(* Logix 5000 AddOnInstructionDefinition export; software revision 16.04 *)

TYPE AKD_Status :   // All connections to the drive ethernet module are established and data is successfully transferring.
STRUCT
   Profile_In_Progress : BOOL;   // Profile Move In Progress
   Block_In_Execution : BOOL;   // Block In Execution
   On_Target_Position : BOOL;   // On Target Position (1=Current Position Equals Last Target Position)
   General_Fault : BOOL;   // General Fault
   Current_Direction : BOOL;   // Current Motor Direction (0=Reverse, 1=Forward)
   Home_Level : BOOL;   // Level of Home Input
   Reg_Level : BOOL;   // Level of Registration Input
   Enable : BOOL;   // State of Enable Output
   Fault_Input_Fault : BOOL;   // Fault Input Active
   Fwd_Limit : BOOL;   // Forward Input Active
   Rev_Limit : BOOL;   // Reverse Input Active
   Positive_Limit : BOOL;   // Positive Software Limit Exceeded
   Negative_Limit : BOOL;   // Negative Software Limit Exceeded
   FE_Fault : BOOL;   // Following Error Fault
   Block_Fault : BOOL;   // Block Execution Fault
   Load_Complete : BOOL;   // Command Message Successfully Loaded
END_STRUCT
END_TYPE

TYPE AKD_Axis :   // Axis Data:
STRUCT
   Control : AKD_Control;   // Control bits to send to the drive
   Status : AKD_Status;   // Status bits received from the drive
   Input : AB:ETHERNET_MODULE_SINT_64Bytes:I:0;   // Data from the drive
   Output : AB:ETHERNET_MODULE_SINT_64Bytes:O:0;   // Data to the drive
   ResponseMsgType : SINT;   // Response type contained in latest IO response from drive. Used to check for errors
   CommandTimeout : INT;   // Time to allow for command response from drive. Dependent on scan rate and communicaiton rate
   PositionFeedback : DINT;   // Actual Position Value
   VelocityFeedback : DINT;   // Actual Velocity Value
END_STRUCT
END_TYPE

TYPE AKD_Control :   // Send Explicit Message
STRUCT
   Load_Data_Start_Profile : BOOL;   // Load Command Data / Start Profile Move
   Start_Block : BOOL;   // Execute Command block or block chain
   Incremental : BOOL;   // Incremental Position (0=Absolute, 1=Incremental)
   Direction : BOOL;   // Direction in Velocity Mode (0=Reverse, 1=Forward)
   Smooth_Stop : BOOL;   // Smooth / Controlled Stop w/ Deceleration
   Hard_Stop : BOOL;   // Hard / Immediate Stop
   Reg_Arm : BOOL;   // Arm the Registration Input
   Enable : BOOL;   // Enable Output
END_STRUCT
END_TYPE

ADD_ON_INSTRUCTION AKD_Disable   (* revision 2.1, ExecutePrescan, ExecuteEnableInFalse *)
// Disable Drive
// Revision note:
// Don't error if Command_Timeout preset is 0
VAR_OUTPUT
   DN : BOOL; {visible}   // Command Successful
   ER : BOOL; {visible}   // Error
END_VAR
VAR_IN_OUT
   Axis : AKD_Axis; {required}
END_VAR
VAR
   Command_Timeout : TIMER;   // Timeout Timer
END_VAR

ROUTINE EnableInFalse   (* ladder *)
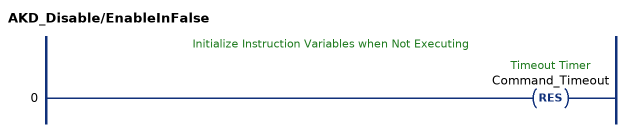
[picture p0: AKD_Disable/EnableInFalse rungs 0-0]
   // Initialize Instruction Variables when Not Executing
   0: RES(Command_Timeout);
END_ROUTINE

ROUTINE Logic   (* ladder *)
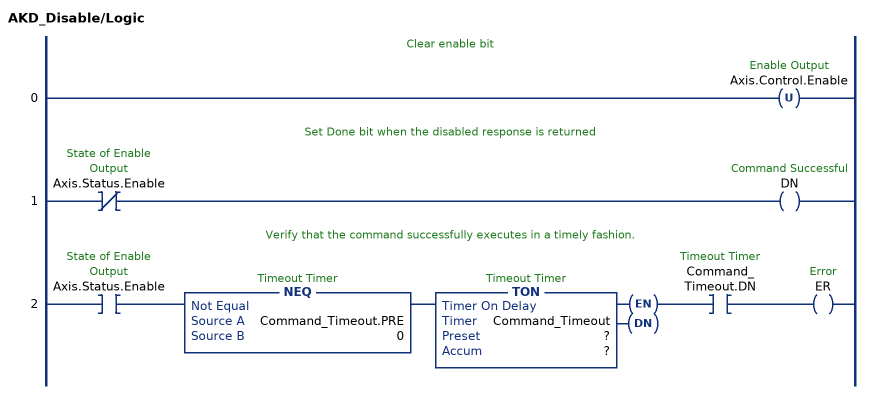
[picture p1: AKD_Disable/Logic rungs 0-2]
   // Clear enable bit
   0: OTU(Axis.Control.Enable);
   // Set Done bit when the disabled response is returned
   1: XIO(Axis.Status.Enable)OTE(DN);
   // Verify that the command successfully executes in a timely fashion.
   2: XIC(Axis.Status.Enable)NEQ(Command_Timeout.PRE,0)TON(Command_Timeout,?,?)XIC(Command_Timeout.DN)OTE(ER);
END_ROUTINE

ROUTINE Prescan   (* ladder *)
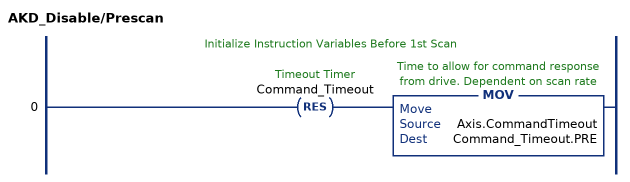
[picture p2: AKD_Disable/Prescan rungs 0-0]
   // Initialize Instruction Variables Before 1st Scan
   0: RES(Command_Timeout)MOV(Axis.CommandTimeout,Command_Timeout.PRE);
END_ROUTINE
END_ADD_ON_INSTRUCTION
